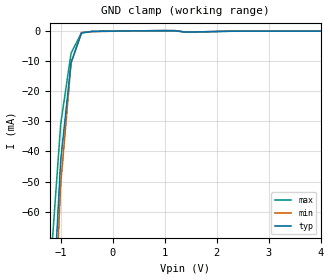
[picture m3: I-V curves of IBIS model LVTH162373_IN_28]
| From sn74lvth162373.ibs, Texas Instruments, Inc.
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|   Model LVTH162373 Input_IN_28
[Model]   LVTH162373_IN_28
Model_type  Input
Polarity   Inverting
Vinl = 0.8V
Vinh = 2.0V
| variable   typ   min   max
C_comp   3p   NA   NA
[Temperature Range]   25   -40   85
[Voltage range]   2.8   2.7   2.9
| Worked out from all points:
|   GND clamp passes 1 mA (typ) near -0.61 V on its own axis
|Process range|   weak   strong
[GND Clamp]
|   Voltage   I(typ)   I(min)   I(max)
-5V       -1.864A    -2.109A    -1.637A
-1.2V     -108.8mA   -129.4mA   -79.42mA
-1V       -43.04mA   -50.99mA   -30.95mA
-800mV    -10.4mA    -10.68mA   -7.349mA
-600mV    -646.2uA   -506.9uA   -521.9uA
-400mV    -100.8uA   -150.6uA   -67.46uA
800mV     156.4uA    170.1uA    150.5uA
1.2V      152.7uA    194.6uA    122.6uA
1.4V      -316.8uA   -322.1uA   -317.4uA
2.2V      -40.03uA   -10.23uA   -60.62uA
5V        -23.02pA   960.2nA    4.768nA
